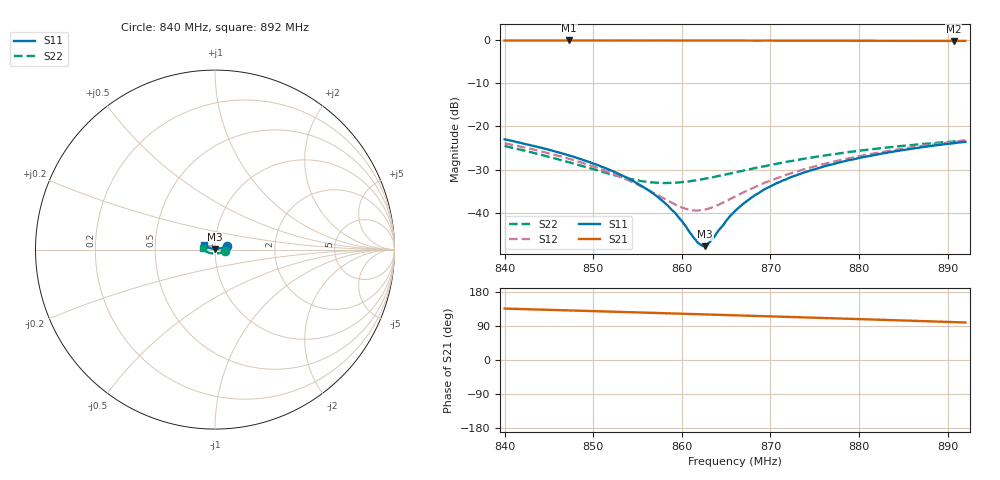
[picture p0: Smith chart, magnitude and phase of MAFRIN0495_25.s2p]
!Part Number:  MAFRIN0495
!Name:  MARIA CRAVEN
!Comments:  1
!Thu 30/Sep/2004  1:52:32 PM
!Temperature:  25
# MHZ  S  DB  R  50
!Freq  S11(dB)  S11(ang)  S21(dB)  S21(ang)  S12(dB)  S12(ang)  S22(dB)  S22(ang)
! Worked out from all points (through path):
!   201 points, 840 MHz to 892 MHz, reference 50 ohm
!   highest |S21| = -0.18 dB at 847.3 MHz (marker M1); lowest = -0.3 dB at 890.7 MHz (marker M2)
!   group delay of S21, straight-line fit = 1.96 ns
!   lowest |S11| = -47.7 dB at 862.6 MHz (marker M3), VSWR 1.01, Z = 50 + j0.41 ohm
!   |S11| at or under -10 dB: start of sweep to end of sweep
!   |S22| runs from -33.1 to -23.3 dB; largest |S21 - S12| = 1
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840  -23.02 15.8  -0.20 135.7  -23.94 94.6  -24.56 -9.3
847.28  -26.76 13.6  -0.18 130.8  -27.53 93.9  -28.33 -27.2
848.84  -27.79 13.3  -0.19 129.8  -28.52 94.4  -29.24 -32.7
851.44  -29.73 13.3  -0.18 128.0  -30.35 96.4  -30.78 -44.3
854.04  -32.15 14.1  -0.19 126.2  -32.56 100.7  -32.11 -58.9
856.38  -34.97 16.5  -0.19 124.6  -34.92 108.5  -32.94 -75.2
857.42  -36.58 18.9  -0.19 123.9  -36.06 113.8  -33.09 -82.7
859.24  -40.01 26.2  -0.20 122.6  -38.07 128.0  -33.05 -96.3
860.54  -43.42 38.6  -0.20 121.8  -39.15 142.8  -32.80 -105.3
861.84  -46.99 66.3  -0.20 120.8  -39.48 160.3  -32.39 -113.9
862.62  -47.71 93.9  -0.20 120.4  -39.26 170.5  -32.14 -118.5
863.66  -45.59 126.0  -0.21 119.6  -38.55 -177.2  -31.72 -124.3
865.22  -41.31 147.7  -0.20 118.5  -37.07 -163.5  -31.04 -131.6
866  -39.59 153.4  -0.21 117.9  -36.26 -158.4  -30.66 -135.0
867.82  -36.53 160.0  -0.21 116.7  -34.45 -150.3  -29.88 -141.9
869.38  -34.51 162.4  -0.21 115.5  -33.03 -145.9  -29.23 -146.8
872.24  -31.83 163.9  -0.23 113.5  -30.93 -141.4  -28.09 -154.4
874.84  -30.02 164.0  -0.23 111.6  -29.35 -139.3  -27.16 -159.9
878.74  -27.89 163.2  -0.24 108.8  -27.46 -138.4  -25.99 -167.1
883.42  -26.02 161.2  -0.26 105.4  -25.68 -138.8  -24.85 -174.2
890.7  -23.92 157.0  -0.29 100.0  -23.61 -141.2  -23.52 176.3
892  -23.61 156.3  -0.29 99.0  -23.31 -141.8  -23.34 174.7
